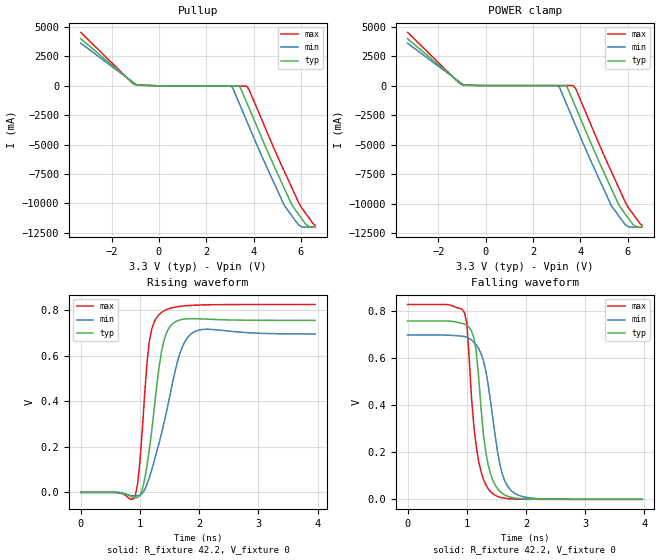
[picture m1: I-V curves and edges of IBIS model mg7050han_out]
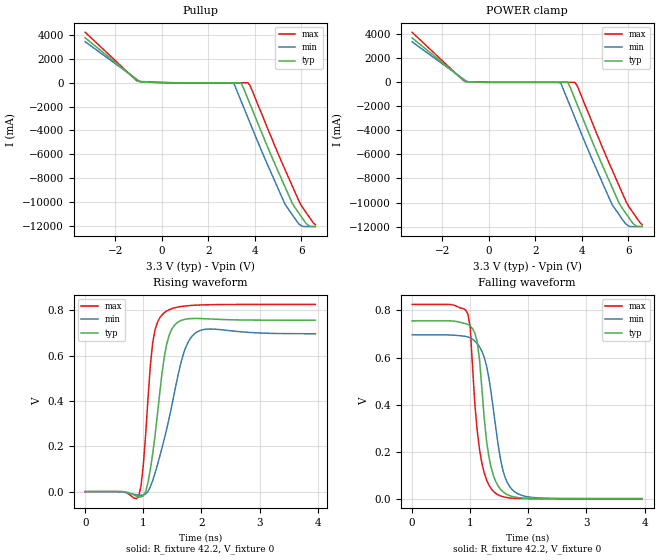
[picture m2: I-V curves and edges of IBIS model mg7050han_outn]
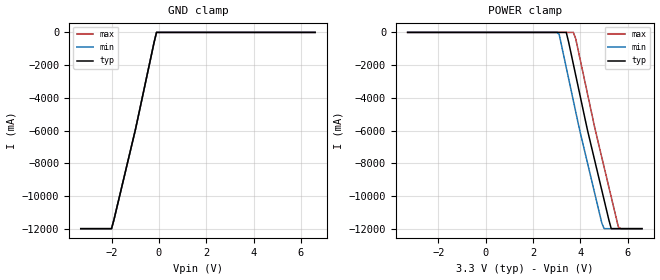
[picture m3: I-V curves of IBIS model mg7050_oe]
|   IBIS File mg7050han_4a_33v_85.ibs  ZSEL=L(ZO=85ohm)
[IBIS Ver]   3.2
[Comment Char]   |_char
[File name]   mg7050han_4a_33v_85.ibs
[File Rev]   1.0
[Date]   Jan 23, 2014
[Source]
|   Component MG7050HAN HCSL 4-OUTPUT 3.3V
[Component]   mg7050han-hcsl-4out-85ohm
[Manufacturer]   Seiko Epson Corporation
[Package]
| variable   typ   min   max
R_pkg   0.27   NA   NA
L_pkg   1.66n   NA   NA
C_pkg   0.53p   NA   NA
[Pin]   signal_name   model_name   R_pin   L_pin   C_pin
1   vcc1   POWER   NA   NA   NA
2   out1p   mg7050han_out   0.34   2.1nH   0.58pF
3   out1n   mg7050han_outn  0.25   1.5nH   0.50pF
4   out2p   mg7050han_out   0.22   1.3nH   0.44pF
5   out2n   mg7050han_outn  0.25   1.7nH   0.59pF
6   zsel   mg7050_zsel   NA   NA   NA
7   oe   mg7050_oe   NA   NA   NA
8   out3n   mg7050han_outn  0.25   1.7nH   0.62pF
9   out3p   mg7050han_out   0.22   1.3nH   0.49pF
10   out4n   mg7050han_outn  0.25   1.5nH   0.46pF
11   out4p   mg7050han_out   0.34   2.1nH   0.57pF
12   vcc2   POWER   NA   NA   NA
13   vcc   POWER   NA   NA   NA
14   gnd   GND   NA   NA   NA
[Diff Pin] inv_pin vdiff   tdelay_typ
2   3   0   0
4   5   0   0
9   8   0   0
11   10   0   0
| Models and submodels in the file (4): mg7050han_out (Open_source), mg7050han_outn (Open_source), mg7050_oe (Input), mg7050_zsel (Input)
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[Model]   mg7050han_out
Model_type Open_source
Enable Active-High
Polarity Non-Inverting
Vref=0
Vmeas=0.375
Rref=42.2
Cref=0
C_comp   4.74p   4.50p   4.98p
[Temperature Range] 25   85   -40
[Voltage Range]   3.3   2.97   3.63
[POWER Clamp Reference]3.3   2.97   3.63
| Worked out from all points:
|   slope of the pullup table from 0 to 0.495 V, typ, clamps not added: 32.1 ohm
|   POWER clamp passes 1 mA (typ) near -0.13 V on its own axis
|   falling waveform, R_fixture 42.2, V_fixture 0: 20-80 % time 189ps typ, 258ps min, 174ps max; typ from 0.756 V to 0 V
|   rising waveform, R_fixture 42.2, V_fixture 0: 20-80 % time 217ps typ, 374ps min, 150ps max; typ from 0 V to 0.756 V
[Pullup]
-3.3V     4.004A     3.625A     4.547A
-1V       106.6mA    168.9mA    95.56mA
3V        -17.96mA   -16.64mA   -19.55mA
3.1V      -17.96mA   -94.24mA   -19.58mA
3.4V      -17.97mA   -1.517A    -19.65mA
3.7V      -1.376A    -2.941A    -19.67mA
3.8V      -1.851A    -3.416A    -285.6mA
5.3V      -8.731A    -10.17A    -7.284A
5.6V      -10.05A    -11.01A    -8.6A
6V        -11.21A    -11.95A    -10.29A
6.3V      -11.91A    -12.02A    -11.12A
6.6V      -12.02A    -12.02A    -11.87A
[POWER Clamp]
-3.3V     3.965A     3.584A     4.513A
-1V       83.27mA    152.1mA    63.84mA
3V        -218.3pA   -251.7pA   -194.6pA
3.1V      -229.5pA   -83.17mA   -205.8pA
3.4V      -263.1pA   -1.507A    -239.5pA
3.7V      -1.364A    -2.93A     -273.1pA
3.8V      -1.839A    -3.405A    -272.9mA
5.3V      -8.719A    -10.16A    -7.271A
5.6V      -10.03A    -11A       -8.587A
6V        -11.19A    -11.94A    -10.27A
6.3V      -11.89A    -12A       -11.11A
6.6V      -12A       -12A       -11.85A
[Falling Waveform]
R_fixture=42.2
V_fixture=0
V_fixture_min=0
V_fixture_max=0
0s        755.8mV    696.3mV    825.7mV
960ps     743.2mV    689.7mV    791.1mV
1ns       737.8mV    686.7mV    746.4mV
1.08ns    712.6mV    675.6mV    427.2mV
1.16ns    625.3mV    654.9mV    222.3mV
1.28ns    277.3mV    588mV      85.3mV
1.44ns    80.34mV    342.1mV    23.69mV
1.6ns     25.01mV    106.3mV    6.489mV
1.84ns    4.559mV    20.98mV    916.3uV
3.96ns    0V         2.569uV    0V
[Rising Waveform]
R_fixture=42.2
V_fixture=0
V_fixture_min=0
V_fixture_max=0
0s        769nV      930.7nV    0V
920ps     -23.59mV   -15.8mV    -17.32mV
1ns       -13.89mV   -12.48mV   137mV
1.12ns    118.6mV    35.64mV    571.6mV
1.16ns    190.5mV    65.83mV    665.3mV
1.36ns    612.1mV    254.3mV    789.8mV
1.48ns    717.4mV    392.7mV    806.3mV
1.64ns    754.8mV    580.4mV    816.1mV
1.88ns    763.5mV    699.7mV    822mV
3.96ns    755.9mV    696.3mV    825.7mV
[Ramp]
R_load=42.2
dV/dt_r   4.535E-1/2.160E-10   4.178E-1/3.732E-10   4.954E-1/1.482E-10
dV/dt_f   4.535E-1/1.875E-10   4.178E-1/2.552E-10   4.954E-1/1.706E-10
|[End   mg7050han_out
[Model]   mg7050han_outn
Model_type Open_source
Enable Active-High
Polarity Inverting
Vref=0
Vmeas=0.375
Rref=42.2
Cref=0
C_comp   4.74p   4.50p   4.98p
[Temperature Range] 25   85   -40
[Voltage Range]   3.3   2.97   3.63
[POWER Clamp Reference]3.3   2.97   3.63
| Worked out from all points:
|   slope of the pullup table from 0 to 0.495 V, typ, clamps not added: 32.1 ohm
|   POWER clamp passes 1 mA (typ) near -0.13 V on its own axis
|   falling waveform, R_fixture 42.2, V_fixture 0: 20-80 % time 191ps typ, 259ps min, 175ps max; typ from 0.756 V to 0 V
|   rising waveform, R_fixture 42.2, V_fixture 0: 20-80 % time 216ps typ, 371ps min, 150ps max; typ from 0 V to 0.756 V
[Pullup]
-3.3V     3.733A     3.407A     4.193A
-1V       102.3mA    158.8mA    94.75mA
3V        -17.96mA   -16.64mA   -19.55mA
3.1V      -17.96mA   -94.24mA   -19.58mA
3.4V      -17.97mA   -1.517A    -19.65mA
3.7V      -1.376A    -2.941A    -19.67mA
3.8V      -1.851A    -3.416A    -285.6mA
5.3V      -8.731A    -10.17A    -7.284A
5.6V      -10.05A    -11.01A    -8.6A
6V        -11.21A    -11.95A    -10.29A
6.3V      -11.91A    -12.02A    -11.12A
6.6V      -12.02A    -12.02A    -11.87A
[POWER Clamp]
-3.3V     3.699A     3.371A     4.162A
-1V       79.56mA    143.1mA    63.14mA
3V        -218.3pA   -251.7pA   -194.7pA
3.1V      -229.5pA   -83.17mA   -205.9pA
3.4V      -263.1pA   -1.507A    -239.5pA
3.7V      -1.364A    -2.93A     -273pA
3.8V      -1.839A    -3.405A    -272.9mA
5.3V      -8.719A    -10.16A    -7.271A
5.6V      -10.03A    -11A       -8.587A
6V        -11.19A    -11.94A    -10.27A
6.3V      -11.9A     -12A       -11.11A
6.6V      -12A       -12A       -11.85A
[Falling Waveform]
R_fixture=42.2
V_fixture=0
V_fixture_min=0
V_fixture_max=0
0s        755.8mV    696.3mV    825.7mV
960ps     740.5mV    687.4mV    785.3mV
1ns       733.8mV    683.4mV    728mV
1.08ns    703.5mV    669.9mV    402mV
1.16ns    591.7mV    645.6mV    209.9mV
1.28ns    247.6mV    565.8mV    80.68mV
1.44ns    72.62mV    301.5mV    22.42mV
1.6ns     22.75mV    90.54mV    6.141mV
1.84ns    4.163mV    18.57mV    866.3uV
3.96ns    0V         2.39uV     0V
[Rising Waveform]
R_fixture=42.2
V_fixture=0
V_fixture_min=0
V_fixture_max=0
0s        -4.027uV   3.371uV    0V
920ps     -23.03mV   -15.47mV   -22.09mV
1ns       -18.57mV   -14.41mV   117.9mV
1.16ns    164.8mV    47.89mV    654.8mV
1.24ns    334.2mV    115.6mV    745.1mV
1.36ns    593.3mV    231.7mV    788.9mV
1.48ns    711.8mV    367.1mV    806mV
1.68ns    757.6mV    599mV      817.5mV
1.92ns    763.6mV    703.7mV    822.5mV
3.96ns    755.9mV    696.4mV    825.7mV
[Ramp]
R_load=42.2
dV/dt_r   4.535E-1/2.146E-10   4.178E-1/3.701E-10   4.954E-1/1.474E-10
dV/dt_f   4.535E-1/1.879E-10   4.178E-1/2.565E-10   4.954E-1/1.711E-10
|[End   mg7050han_outn
[Model]   mg7050_oe
Model_type Input
Vinh=2.31
Vinl=0.99
C_comp   3p   3p   3p
[Temperature Range] 25   85   -40
[Voltage Range]   3.3   2.97   3.63
[POWER Clamp Reference]3.3   2.97   3.63
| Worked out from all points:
|   GND clamp passes 1 mA (typ) near -0.10 V on its own axis
[GND Clamp]
-3.3V     -12A       -12A       -12A
-2V       -12A       -12A       -12A
-1.9V     -11.47A    -11.47A    -11.47A
-1V       -6A        -6A        -6A
-200mV    -592.5mA   -592.5mA   -592.5mA
-100mV    -33.15uA   -29.16uA   -40.33uA
6.6V      32.19uA    34.53uA    32.12uA
[POWER Clamp]
-3.3V     32.19uA    31.39uA    35.69uA
3V        -29.25uA   -28.49uA   -32.44uA
3.1V      -30.22uA   -118.5mA   -33.52uA
3.4V      -33.15uA   -2.15A     -36.76uA
3.7V      -1.947A    -4.181A    -40uA
3.8V      -2.624A    -4.859A    -389.4mA
4.3V      -6A        -8.004A    -3.775A
4.9V      -9.645A    -11.65A    -7.64A
5V        -10.25A    -12A       -8.248A
5.3V      -12A       -12A       -10.07A
5.6V      -12A       -12A       -11.89A
6.6V      -12A       -12A       -12A
